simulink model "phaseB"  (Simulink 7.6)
settings: Solver=ode23tb  StartTime=0.0  StopTime=0.02  RelTol=1e-3
InitFcn:
  | clear all
  | close all
  | clc
  | delete *.mat
StopFcn:
  | load phaseB.mat
  | plot(x(1,:),x(2,:),x(1,:),x(3,:))
  | grid
  | title('Tension d''entrée et de sortie - Phase B')
  | xlabel('temps')
  | axis([0 0.02 -2 12])
  | 
  | delete *.mat
libraries: powerlib x8

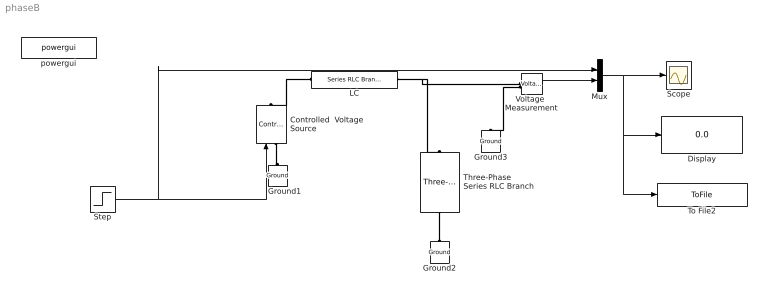
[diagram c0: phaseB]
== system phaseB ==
  Controlled  Voltage Source : powerlib/Electrical Sources/Controlled Voltage Source  DialogController=POWERSYS.PowerSysDialog  SystemSampleTime=-1  Initialize=on  Source_Type=AC  Amplitude=0  Phase=0  Frequency=0  Measurements=None
  Display : Display
  Ground1 : powerlib/Elements/Ground  DialogController=POWERSYS.PowerSysDialog  PhysicalDomain=powersysdomain  SubClassName=unknown  LeftPortType=p1  RightPortType=p1  LConnTagsString=a
  Ground2 : powerlib/Elements/Ground  DialogController=POWERSYS.PowerSysDialog  PhysicalDomain=powersysdomain  SubClassName=unknown  LeftPortType=p1  RightPortType=p1  LConnTagsString=a
  Ground3 : powerlib/Elements/Ground  DialogController=POWERSYS.PowerSysDialog  PhysicalDomain=powersysdomain  SubClassName=unknown  LeftPortType=p1  RightPortType=p1  LConnTagsString=a
  LC : powerlib/Elements/Series RLC Branch  DialogController=POWERSYS.PowerSysDialog  PhysicalDomain=powersysdomain  SubClassName=unknown  LeftPortType=p1  RightPortType=p1  LConnTagsString=__new0  RConnTagsString=__new0  BranchType=LC  Resistance=10  Inductance=0.001  SetiL0=off  InitialCurrent=0  Capacitance=1e-3  Setx0=off  InitialVoltage=0  Measurements=None
  Mux : Mux  Inputs=2
  Scope : Scope
  Step : Step  Time=0.005  After=10  SampleTime=0
  Three-Phase Series RLC Branch : powerlib/Elements/Three-Phase Series RLC Branch  DialogController=POWERSYS.PowerSysDialog  PhysicalDomain=powersysdomain  SubClassName=unknown  LeftPortType=p1  RightPortType=p1  LConnTagsString=A|B|C  RConnTagsString=A|B|C  BranchType=R  Resistance=1  Inductance=1e-3  Capacitance=1e-6  Measurements=None
  To File2 : ToFile  Filename=phaseB  MatrixName=x
  Voltage  Measurement : powerlib/Measurements/Voltage Measurement  DialogController=POWERSYS.PowerSysDialog  SystemSampleTime=-1  PhasorSimulation=off  OutputType=Complex  PSBequivalent=0
  powergui : powerlib/powergui  Priority=2  SystemSampleTime=-1  SimulationMode=Continuous  SampleTime=0  frequency=60  SPID=off  DisableSnubberDevices=off  DisableRonSwitches=off  DisableVfSwitches=off  SwTol=0  Interpol=off  frequencyindice=0  echomessages=off  HookPort=off  DisplayEquations=off  FunctionMessages=off  EnableUseOfTLC=off  x0status=blocks  RestoreLinks=warning  ResistiveCurrentMeasurement=off  Frange=logspace(0,3,50)  Ylog=off  Xlog=off  ShowGrid=off  save=off  variable=ZData  ZoomFFT=on  StartTime=0.0  cycles=1  DisplayStyle=off  fundamental=60  FreqAxis=off  MaxFrequency=1000  frequencyindicesteady=1  RmsSteady=1  display=off  Ts=0  methode=off
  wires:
  Step/1 -> Controlled  Voltage Source/1, Mux/1
  Voltage  Measurement/1 -> Mux/2
  Mux/1 -> Scope/1, Display/1, To File2/1
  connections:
  Controlled  Voltage Source/LConn1 -- Ground1/LConn1
  LC/RConn1 -- Three-Phase Series RLC Branch/RConn2 -- Voltage  Measurement/LConn1
  LC/LConn1 -- Controlled  Voltage Source/RConn1
  Three-Phase Series RLC Branch/LConn2 -- Ground2/LConn1
  Voltage  Measurement/LConn2 -- Ground3/LConn1
